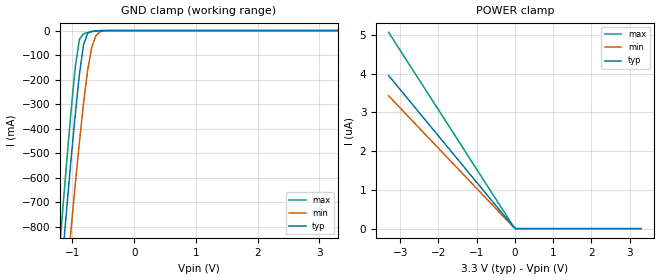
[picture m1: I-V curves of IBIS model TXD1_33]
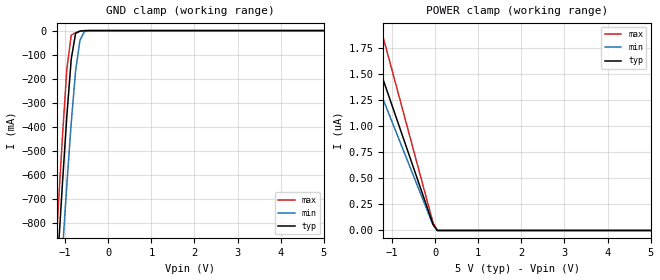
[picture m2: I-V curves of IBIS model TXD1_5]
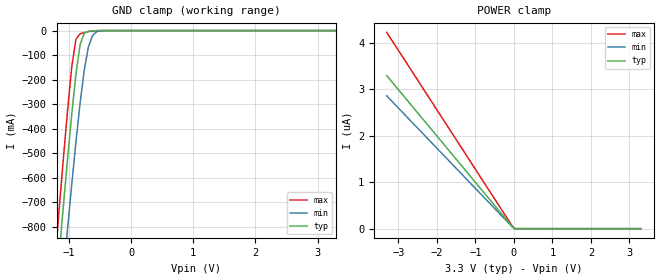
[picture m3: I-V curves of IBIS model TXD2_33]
| IBIS file created by Layout Workbench Version 22.1.4.12161.401368   004
| Cadence Design Systems, Inc. 2011
[IBIS ver]   4.2
[File name]  isow6441.ibs
[File Rev]   1.0
[Date]   03 26, 2026
[Source]   Model built from TISPICED simulations at:
   Texas Instruments Incorporated.
   Analog-eLab, HPA 12500 TI Blvd
   Dallas, TX -75243
   For Support e-mail: elab_ibis@list.ti.com
[Notes]   This product is designed as an aid for customers of Texas Instruments.
   No warranties, either expressed or implied, with respect to this third party software (if any)
   or with respect to its fitness for any particular purpose is claimed by Texas Instruments or
   the author. The software (if any) is provided solely on an "as is" basis. The entire risk as to
   its quality and performance is with the customer
[Disclaimer]  This product is designed as an aid for customers of Texas Instruments. No warranties, either expressed or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
[Copyright] (C)Copyright 2025 Texas Instruments Incorporated. All rights reserved.
|   Component ISO64XX
[Component] ISOW6441DW
[Manufacturer] Texas Instruments Incorporated
[Package]   |16-pin SOIC DW package
|   typ   min   max
R_pkg   0.04817   0.03432   0.09530
L_pkg   2.4595nH   1.6904nH   4.7034nH
C_pkg   0.847pF   0.428pF   1.397pF
[Pin]  signal_name   model_name   R_pin   L_pin   C_pin
1   VCC1   POWER   0.03455  3.39778n  0.89677p
2   GND1   GND   0.03432  3.12613n  0.84706p
3   INA   TXD1   0.04265  1.85523n  0.57831p
4   INB   TXD2   0.03948  1.69049n  0.59300p
5   INC   TXD2   0.06147  2.13194n  0.42769p
6   OUTD   RXD1   0.04257  1.86953n  0.56379p
7   NC   NC   0.04783  1.99000n  0.60148p
8   GND1   GND   0.03740  4.70338n  1.39696p
9   GND2   GND   0.03763  4.61305n  1.39587p
10   SEL   TXDM1   0.04703  2.01514n  0.58483p
11   IND   TXD2   0.07132  2.45946n  0.43321p
12   OUTC   RXD1   0.03943  1.70546n  0.55709p
13   OUTB   RXD1   0.07288  2.39260n  0.48001p
14   OUTA   RXD1   0.09530  3.03704n  0.47622p
15   GND2   GND   0.04817  4.23145n  0.93567p
16   VCC2   POWER   0.04790  4.51154n  0.99405p
[Model Selector] TXD1
TXD1_33   TXD Input model for 3.0V - 3.6V
TXD1_5   TXD Input model for 4.5V - 5.5V
[Model Selector] RXD1
RXD_33   RXD Output model for 3.0V - 3.6V
RXD_5   RXD Output model for 4.5V - 5.5V
[Model Selector] TXDM1
TXDM_33   TXD Input model for 3.0V - 3.6V
TXDM_5   TXD Input model for 4.5V - 5.5V
[Model Selector] TXD2
TXD2_33   TXD Input model for 3.0V - 3.6V
TXD2_5   TXD Input model for 4.5V - 5.5V
| Models and submodels in the file (8): TXD1_33 (Input), TXD1_5 (Input), TXD2_33 (Input), TXD2_5 (Input), TXDM_33 (Input), TXDM_5 (Input), RXD_33 (3-state), RXD_5 (3-state)
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|   TXD1_33 Model
[Model]   TXD1_33
Model_type Input
Polarity   Non-Inverting
Enable   Active-High
Vinl =  0.990V
Vinh =  2.310V
C_comp   1.300pF   1.100pF   1.500pF
[Model Spec]
Vinh   2.310V   2.079V   2.541V
Vinl   0.990V   0.891V   1.089V
[Temperature Range]   27.000   0.150k   -55.000
[Voltage Range]   3.300V   3.000V   3.600V
[POWER Clamp Reference]   3.300V   3.000V   3.600V
[GND Clamp Reference]   0.0V   0.0V   0.0V
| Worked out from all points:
|   GND clamp passes 1 mA (typ) near -0.62 V on its own axis
[GND_clamp]
|Voltage   I(typ)   I(min)   I(max)
-3.3V     -6.511A    -6.3A      -6.742A
-1.223V   -1.108A    -1.374A    -932.4mA
-1.156V   -908.9mA   -1.182A    -724.2mA
-1.089V   -712.9mA   -993.1mA   -520.4mA
-1.022V   -522.3mA   -807.7mA   -324.9mA
-955mV    -341.3mA   -627.5mA   -147.8mA
-888mV    -178.8mA   -455.4mA   -35.62mA
-821mV    -57.82mA   -296.5mA   -13.04mA
-754mV    -10.68mA   -161mA     -8.05mA
-687mV    -2.941mA   -66.52mA   -4.244mA
-553mV    -287.9uA   -4.329mA   -378.7uA
3.3V      0A         0A         -460.3nA
[POWER_clamp]
|Voltage   I(typ)   I(min)   I(max)
-3.3V     3.95uA     3.427uA    5.064uA
-50mV     59.91nA    53.72nA    76.8nA
17mV      0A         0A         0A
3.3V      0A         0A         0A
|   TXD1_5 Model
[Model]   TXD1_5
Model_type Input
Polarity   Inverting
Enable   Active-High
Vinl =  1.500V
Vinh =  3.500V
C_comp   1.300pF   1.100pF   1.500pF
[Model Spec]
Vinh   3.500V   3.150V   3.850V
Vinl   1.500V   1.350V   1.650V
[Temperature Range]   27.000   0.150k   -55.000
[Voltage Range]   5.000V   4.500V   5.500V
[POWER Clamp Reference]   5.000V   4.500V   5.500V
[GND Clamp Reference]   0.0V   0.0V   0.0V
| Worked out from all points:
|   GND clamp passes 1 mA (typ) near -0.60 V on its own axis
[GND_clamp]
|Voltage   I(typ)   I(min)   I(max)
-5V       -9.985A    -9.609A    -10.4A
-1.263V   -1.229A    -1.49A     -1.058A
-1.162V   -926.6mA   -1.199A    -742.7mA
-1.061V   -632.4mA   -915.1mA   -437.4mA
-960mV    -354.3mA   -640.8mA   -159.9mA
-859mV    -119.3mA   -384.6mA   -19.73mA
-758mV    -11.77mA   -168.2mA   -8.316mA
-657mV    -1.875mA   -40.74mA   -2.94mA
-556mV    -310.1uA   -4.661mA   -414.1uA
-455mV    -23.79uA   -355uA     -18.34uA
5V        0A         0A         -767.5nA
[POWER_clamp]
|Voltage   I(typ)   I(min)   I(max)
-5V       5.989uA    5.198uA    7.677uA
-1.868V   2.237uA    1.943uA    2.868uA
-1.767V   2.116uA    1.838uA    2.713uA
-1.666V   1.995uA    1.733uA    2.558uA
-1.565V   1.875uA    1.628uA    2.403uA
-1.262V   1.512uA    1.313uA    1.938uA
-1.161V   1.391uA    1.208uA    1.782uA
-50mV     59.98nA    53.97nA    76.87nA
51mV      0A         0A         0A
5V        0A         0A         0A
|   TXD2_33 Model
[Model]   TXD2_33
Model_type Input
Polarity   Non-Inverting
Enable   Active-High
Vinl =  0.990V
Vinh =  2.310V
C_comp   1.300pF   1.100pF   1.500pF
[Model Spec]
Vinh   2.310V   2.079V   2.541V
Vinl   0.990V   0.891V   1.089V
[Temperature Range]   27.000   0.150k   -55.000
[Voltage Range]   3.300V   3.000V   3.600V
[POWER Clamp Reference]   3.300V   3.000V   3.600V
[GND Clamp Reference]   0.0V   0.0V   0.0V
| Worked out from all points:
|   GND clamp passes 1 mA (typ) near -0.62 V on its own axis
[GND_clamp]
|Voltage   I(typ)   I(min)   I(max)
-3.3V     -6.509A    -6.298A    -6.74A
-1.223V   -1.108A    -1.373A    -931.9mA
-1.156V   -908.4mA   -1.182A    -723.7mA
-1.089V   -712.5mA   -992.7mA   -520mA
-1.022V   -522mA     -807.3mA   -324.5mA
-955mV    -341.1mA   -627.2mA   -147.5mA
-888mV    -178.6mA   -455.1mA   -35.36mA
-821mV    -57.67mA   -296.2mA   -12.84mA
-754mV    -10.57mA   -160.9mA   -7.896mA
-687mV    -2.867mA   -66.39mA   -4.141mA
-553mV    -271.5uA   -4.282mA   -357.9uA
3.3V      0A         0A         -383.6nA
[POWER_clamp]
|Voltage   I(typ)   I(min)   I(max)
-3.3V     3.291uA    2.856uA    4.22uA
-50mV     49.89nA    44.91nA    63.98nA
17mV      0A         0A         0A
3.3V      0A         0A         0A
